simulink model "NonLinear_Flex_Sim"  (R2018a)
settings: Solver=ode3  StartTime=0.0  StopTime=10000  FixedStep=Ts  MaxStep=0.5  RelTol=1e-3  EnableMultiTasking=on
InitFcn:
  | run
StopFcn:
  | pl
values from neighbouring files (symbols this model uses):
  Cw2b = [ 0,          0,          0    [run.m]
  d2r = pi/180    (= 0.0174532925199)    [run.m]    (also in runf.m; orbitic.m; Quan.m)
  Hco = [Hy0, 0, 0]'    [run.m]
  ini = [wb0; atto; Hco]    [run.m]
  Kq1 = I22*ww^2 - 3*wo2*(I11-I33)    [run.m]
  Kq2 = 2*I22*zet*ww    [run.m]
  Kqi = 0.0005    [run.m]
  Kr1 = (0.1*I11*I33*zet^2/Hy0) - sqrt( ((0.01^zet^4*I11^2*I33^2)/Hy0^2)+(4*I11*I33*zet^2) )    [run.m]
  Kr2 = 0.05*Kr1    [run.m]
  Kr3 = 0.04*zet*(Kr2-Hy0) * sqrt(abs(Hy0/(I11*I33)))    [run.m]
  nt = 7    [run.m]    (also in runf.m)
  Tmax = 0.05    [run.m]
  Ts = 0.001    [run.m]    (also in runf.m = 0.0005)
  wb0 = [0.0, -wo, 0.0]'    [run.m]
  wo = Worb    [run.m]
  wr0 = [-500.0, 0.0, 0.0]    [run.m]
undefined symbols (not defined in the file or in its folder): Avf, Bvf, Cvf, den, DiscIntNeverNeededParam, Dvf, Mode_Switch, num, Phase_Plane, RW_Steering, Spacecraft_Dynamics, Wheel_Dynamics
libraries: simulink x4

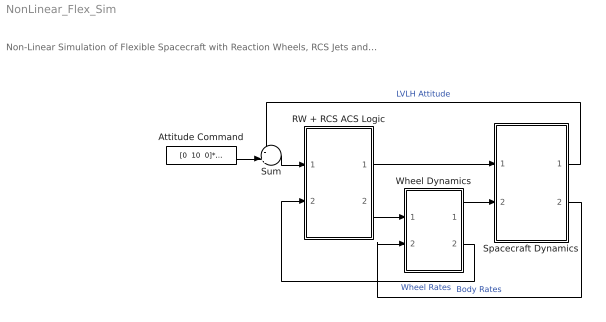
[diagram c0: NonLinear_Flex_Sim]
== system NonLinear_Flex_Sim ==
  note: Non-Linear Simulation of Flexible Spacecraft with Reaction Wheels, RCS Jets and Momentum Bias
  Attitude Command : Constant  Value="[0  10  0]*d2r"
  RW + RCS ACS Logic : Subsystem
  Spacecraft Dynamics : Subsystem
  Sum : Sum  Inputs=-+|
  Wheel Dynamics : Subsystem
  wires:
  Attitude Command/1 -> Sum/2
  Sum/1 -> RW + RCS ACS Logic/1(atter)
  Wheel Dynamics/2(wr) -> RW + RCS ACS Logic/2(wr(i))  "Wheel Rates"
  RW + RCS ACS Logic/2(Trwi) -> Wheel Dynamics/1(Twi)
  Spacecraft Dynamics/1(atti) -> Sum/1  "LVLH Attitude"
  Spacecraft Dynamics/2(wb) -> Wheel Dynamics/2(wb)  "Body Rates"
  RW + RCS ACS Logic/1(Frcs) -> Spacecraft Dynamics/1(Frcs)
  Wheel Dynamics/1(Tcb) -> Spacecraft Dynamics/2(Trwa)

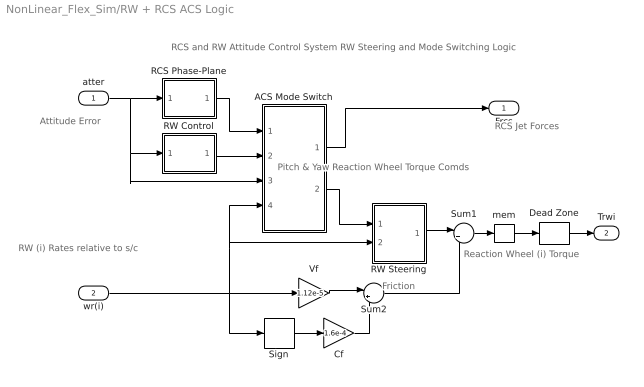
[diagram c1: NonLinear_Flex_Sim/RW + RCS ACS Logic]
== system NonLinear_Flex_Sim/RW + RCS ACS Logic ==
  note: Reaction Wheel (i) Torque
  note: RW (i) Rates relative to s/c
  note: Attitude Error
  note: Pitch & Yaw Reaction Wheel Torque Comds
  note: Friction
  note: RCS Jet Forces
  note: RCS and RW Attitude Control System RW Steering and Mode Switching Logic
  atter : Inport
  wr(i) : Inport  Port=2
  ACS Mode Switch : Subsystem
  Cf : Gain  Gain=1.6e-4
  Dead Zone : DeadZone  LowerValue=-[1, 1, 1]*Tmax/1000  UpperValue=[1 1 1]*Tmax/1000
  RCS Phase-Plane : Subsystem
  RW Control : Subsystem
  RW Steering : Subsystem
  Sign : Signum
  Sum1 : Sum  Inputs=|+-
  Sum2 : Sum  Inputs=|++
  Vf : Gain  Gain=1.12e-5
  mem : Memory  InheritSampleTime=on
  Frcs : Outport
  Trwi : Outport  Port=2
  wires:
  atter/1 -> RCS Phase-Plane/1(atter), ACS Mode Switch/3(atter), RW Control/1(atti)
  RW Control/1(Tc) -> ACS Mode Switch/2(Trw)
  RCS Phase-Plane/1(f(nt)) -> ACS Mode Switch/1(Frcs)
  ACS Mode Switch/2(" Trw") -> RW Steering/1(Trwc)
  ACS Mode Switch/1(" Frcs") -> Frcs/1
  RW Steering/1(Twic) -> Sum1/1
  Sum1/1 -> mem/1
  Dead Zone/1 -> Trwi/1
  Cf/1 -> Sum2/2
  Vf/1 -> Sum2/1
  Sign/1 -> Cf/1
  Sum2/1 -> Sum1/2
  mem/1 -> Dead Zone/1
  wr(i)/1 -> ACS Mode Switch/4(wr(i)), RW Steering/2(wr(1)), Sign/1, Vf/1

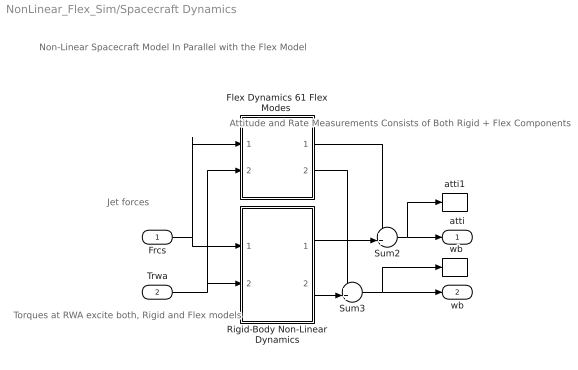
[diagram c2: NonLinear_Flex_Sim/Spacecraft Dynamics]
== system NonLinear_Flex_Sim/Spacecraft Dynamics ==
  note: Non-Linear Spacecraft Model In Parallel with the Flex Model
  note: Torques at RWA excite both, Rigid and Flex models
  note: Jet forces
  note: Attitude and Rate Measurements Consists of Both Rigid + Flex Components
  Frcs : Inport
  Trwa : Inport  Port=2
  "  wb " : ToWorkspace  VariableName=wb  SampleTime=-1
  "Flex Dynamics 61 Flex Modes " : Subsystem
  Rigid-Body Non-Linear Dynamics : Subsystem
  Sum2 : Sum  Inputs=++|
  Sum3 : Sum  Inputs=++|
  atti1 : ToWorkspace  VariableName=atti  SampleTime=-1
  atti : Outport
  wb : Outport  Port=2
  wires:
  Frcs/1 -> "Flex Dynamics 61 Flex Modes "/1(Frcs), Rigid-Body Non-Linear Dynamics/1(Frcs)
  Trwa/1 -> "Flex Dynamics 61 Flex Modes "/2(Trwi), Rigid-Body Non-Linear Dynamics/2(Tcb)
  "Flex Dynamics 61 Flex Modes "/1(att-flx) -> Sum2/1
  Rigid-Body Non-Linear Dynamics/1(atti) -> Sum2/2
  Rigid-Body Non-Linear Dynamics/2(wbr) -> Sum3/2
  "Flex Dynamics 61 Flex Modes "/2(wb-flx) -> Sum3/1
  Sum2/1 -> atti/1, atti1/1
  Sum3/1 -> wb/1, "  wb "/1

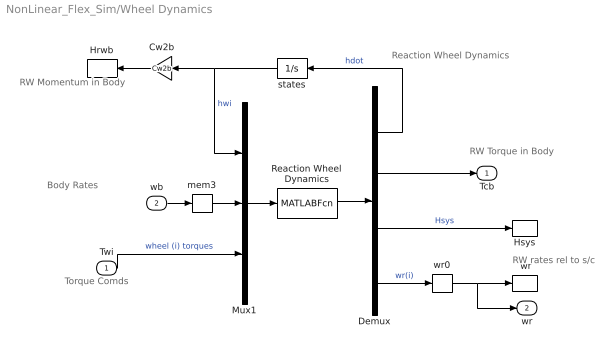
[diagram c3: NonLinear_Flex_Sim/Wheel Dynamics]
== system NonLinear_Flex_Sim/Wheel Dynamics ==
  note: Reaction Wheel Dynamics
  note: Body Rates
  note: RW Torque in Body
  note: RW rates rel to s/c
  note: Torque Comds
  note: RW Momentum in Body
  Twi : Inport
  wb : Inport  Port=2
  " wr" : ToWorkspace  VariableName=wr  SampleTime=-1
  Cw2b : Gain  Gain=Cw2b  Multiplication=Matrix(K*u)
  Demux : Demux  Outputs=[3, 3, 3, 3]
  Hrwb : ToWorkspace  VariableName=Hrwb  SampleTime=-1
  Hsys : ToWorkspace  VariableName=Hsys  SampleTime=-1
  Mux1 : Mux  Inputs=[3, 3, 3]
  Reaction Wheel Dynamics : MATLABFcn  MATLABFcn=Wheel_Dynamics( u(1:3), u(4:6), u(7:9) )  OutputDimensions=3+3+3+3
  mem3 : Memory  InitialCondition=wb0  InheritSampleTime=on
  states : Integrator  InitialCondition=Hco
  wr0 : Memory  InitialCondition=wr0  InheritSampleTime=on
  Tcb : Outport
  wr : Outport  Port=2
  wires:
  states/1 -> Cw2b/1, Mux1/1  "hwi"
  Cw2b/1 -> Hrwb/1
  Demux/1 -> states/1  "hdot"
  Demux/3 -> Hsys/1  "Hsys"
  Demux/4 -> wr0/1  "wr(i)"
  wb/1 -> mem3/1
  Mux1/1 -> Reaction Wheel Dynamics/1
  Reaction Wheel Dynamics/1 -> Demux/1
  Demux/2 -> Tcb/1
  Twi/1 -> Mux1/3  "wheel (i) torques"
  mem3/1 -> Mux1/2
  wr0/1 -> " wr"/1, wr/1

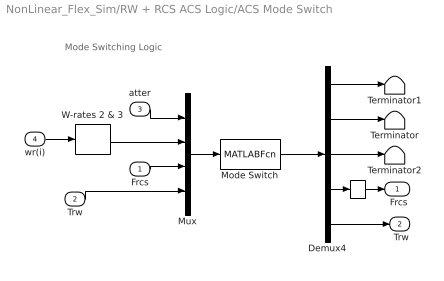
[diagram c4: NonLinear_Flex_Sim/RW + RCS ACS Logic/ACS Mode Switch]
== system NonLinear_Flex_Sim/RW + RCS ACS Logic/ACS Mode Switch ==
  note: Mode Switching Logic
  Frcs : Inport
  Trw : Inport  Port=2
  atter : Inport  Port=3
  wr(i) : Inport  Port=4
  "   " : Memory
  Demux4 : Demux  Outputs="[1 1 1 nt  2]"
  Mode Switch : MATLABFcn  MATLABFcn=Mode_Switch( u(1:3), u(4:5), u(6:5+nt), u(6+nt:7+nt) )  OutputDimensions=3+nt+2
  Mux : Mux  Inputs="[3  2  nt 2]"
  Terminator : Terminator
  Terminator1 : Terminator
  Terminator2 : Terminator
  W-rates 2 & 3 : Selector  InputPortWidth=3  IndexOptions=Index vector (dialog)  Indices="[2  3]"  OutputSizes=1
  " Frcs" : Outport
  " Trw" : Outport  Port=2
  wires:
  atter/1 -> Mux/1
  Mux/1 -> Mode Switch/1
  wr(i)/1 -> W-rates 2 & 3/1
  Frcs/1 -> Mux/3
  Trw/1 -> Mux/4
  Mode Switch/1 -> Demux4/1
  Demux4/4 -> "   "/1
  Demux4/5 -> " Trw"/1
  "   "/1 -> " Frcs"/1
  W-rates 2 & 3/1 -> Mux/2
  Demux4/1 -> Terminator1/1
  Demux4/2 -> Terminator/1
  Demux4/3 -> Terminator2/1

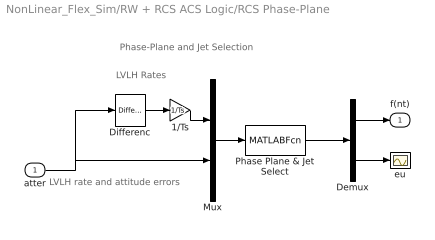
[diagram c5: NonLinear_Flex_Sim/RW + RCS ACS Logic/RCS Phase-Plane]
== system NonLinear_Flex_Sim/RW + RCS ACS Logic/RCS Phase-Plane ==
  note: LVLH rate and attitude errors
  note: LVLH Rates
  note: Phase-Plane and Jet Selection
  atter : Inport
  1/Ts : Gain  Gain=1/Ts
  Demux : Demux  Outputs=[nt, 3]
  Differenc : simulink/Discrete/Difference  ICPrevInput=0.0  InputProcessing=Inherited  OutMin=[]  OutMax=[]  OutDataType=sfix(16)  OutScaling=2^-10  DoSatur=off
  Mux : Mux  Inputs="[3  3]"
  Phase Plane & Jet Select : MATLABFcn  MATLABFcn=Phase_Plane( u(1:3), u(4:6) )  OutputDimensions=nt + 3
  eu : Scope
  f(nt) : Outport
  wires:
  atter/1 -> Mux/2, Differenc/1
  1/Ts/1 -> Mux/1
  Demux/2 -> eu/1
  Demux/1 -> f(nt)/1
  Phase Plane & Jet Select/1 -> Demux/1
  Mux/1 -> Phase Plane & Jet Select/1
  Differenc/1 -> 1/Ts/1

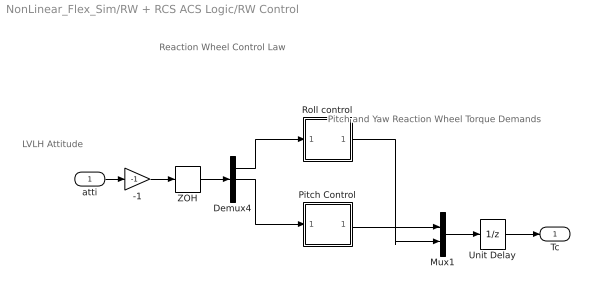
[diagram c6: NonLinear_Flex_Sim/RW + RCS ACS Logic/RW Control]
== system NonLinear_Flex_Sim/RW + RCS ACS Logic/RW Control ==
  note: Pitch and Yaw Reaction Wheel Torque Demands
  note: LVLH Attitude
  note: Reaction Wheel Control Law
  atti : Inport
  -1 : Gain  Gain=-1
  Demux4 : Demux  Outputs=3
  Mux1 : Mux  Inputs=2
  Pitch Control : Subsystem
  Roll control : Subsystem
  Unit Delay : UnitDelay  SampleTime=-1
  ZOH : ZeroOrderHold  SampleTime=Ts
  Tc : Outport
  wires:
  Demux4/1 -> Roll control/1(phi)
  Pitch Control/1(Tcy) -> Mux1/1
  Demux4/2 -> Pitch Control/1(the)
  atti/1 -> -1/1
  Roll control/1(Tcz) -> Mux1/2
  Mux1/1 -> Unit Delay/1
  ZOH/1 -> Demux4/1
  -1/1 -> ZOH/1
  Unit Delay/1 -> Tc/1

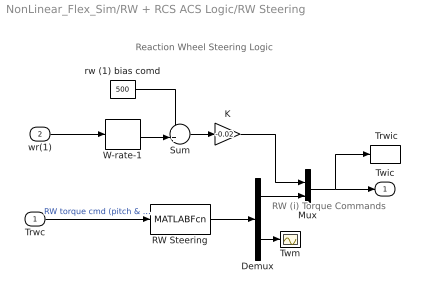
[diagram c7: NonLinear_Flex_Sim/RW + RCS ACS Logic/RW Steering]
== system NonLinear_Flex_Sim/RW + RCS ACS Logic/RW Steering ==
  note: RW (i) Torque Commands
  note: Reaction Wheel Steering Logic
  Trwc : Inport
  wr(1) : Inport  Port=2
  " Trwic" : ToWorkspace  VariableName=Twic  SampleTime=-1
  Demux : Demux  Outputs=[2, 1]
  K : Gain  Gain=-0.02
  Mux : Mux  Inputs=[1,2]
  RW Steering : MATLABFcn  MATLABFcn=RW_Steering( u(1:2) )  OutputDimensions=3
  Sum : Sum  Inputs=++|
  Twm : Scope
  W-rate-1 : Selector  InputPortWidth=3  IndexOptions=Index vector (dialog)  Indices=[1]  OutputSizes=1
  rw (1) bias comd : Constant  Value=500
  Twic : Outport
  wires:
  Demux/2 -> Twm/1
  Demux/1 -> Mux/2
  RW Steering/1 -> Demux/1
  Trwc/1 -> RW Steering/1  "RW torque cmd (pitch & yaw)"
  wr(1)/1 -> W-rate-1/1
  Sum/1 -> K/1
  rw (1) bias comd/1 -> Sum/1
  W-rate-1/1 -> Sum/2
  K/1 -> Mux/1
  Mux/1 -> Twic/1, " Trwic"/1

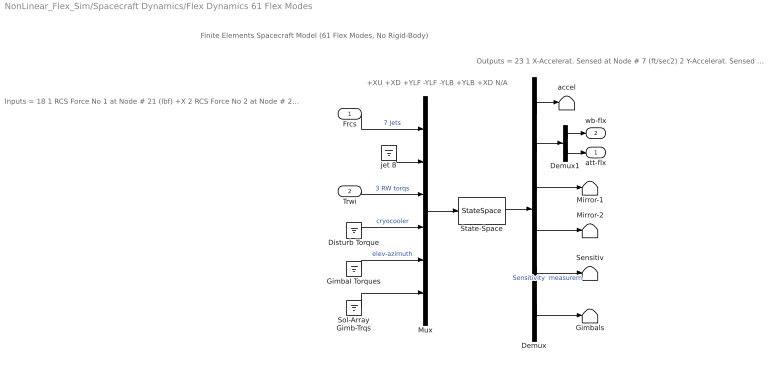
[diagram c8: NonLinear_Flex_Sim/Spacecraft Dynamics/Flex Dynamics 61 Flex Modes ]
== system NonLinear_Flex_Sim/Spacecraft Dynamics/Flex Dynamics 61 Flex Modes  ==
  note: +XU +XD +YLF -YLF -YLB +YLB +XD N/A
  note: Outputs = 23 1 X-Accelerat. Sensed at Node # 7 (ft/sec2) 2 Y-Accelerat. Sensed at Node # 7 (ft/sec2) 3 X-Rot. Rate Sensed at Node # 6 (radian) 4 Y-Rot. Rate Sensed at Node # 6 (radian) 5 Z-Rot. Rate Sensed at Node # 6 (radian) 6 X-Rotation Sensed at Node # 6 (radian) 7 Y-Rotation Sensed at Node # 6 (radian) 8 Z-Rotation Sensed at Node # 6 (radian) 9 Y-Rotation Mirror at Node # 9 (radian) 10 Z-Rotation Mirror at Node # 9 (radian) 11 Y-Rotation Instrum-2 Node # 10 (radian) 12 Z-Rotation Instrum-2 Node # 10 (radian) 13 X-Rotation Instrum-3 Node # 11 (radian) 14 Y-Rotation Instrum-4 Node # 12 (radian) 15 Z-Rotation Instrum-5 Node # 13 (radian) 16 Rotation Angle at Elevati Gimbal No 1 17 Rotation Rate at Elevati Gimbal No 1 18 Rotation Angle at Azimuth Gimbal No 2 19 Rotation Rate at Azimuth Gimbal No 2 20 Rotation Angle at Rght SA Gimbal No 3 21 Rotation Rate at Rght SA Gimbal No 3 22 Rotation Angle at Left SA Gimbal No 4 23 Rotation Rate at Left SA Gimbal No 4
  note: Inputs = 18 1 RCS Force No 1 at Node # 21 (lbf) +X 2 RCS Force No 2 at Node # 22 (lbf) +X 3 RCS Force No 3 at Node # 23 (lbf) +Y 4 RCS Force No 4 at Node # 24 (lbf) -Y 5 RCS Force No 5 at Node # 25 (lbf) -Y 6 RCS Force No 6 at Node # 26 (lbf) +Y 7 RCS Force No 7 at Node # 27 (lbf) +X 8 RCS Force No 8 at Node # 28 (lbf) +X 9 RW Torque No 1 at Node # 17 (ft-lb) roll 10 RW Torque No 2 at Node # 18 (ft-lb) ptch 11 RW Torque No 3 at Node # 19 (ft-lb) yaw 12 Dist Trque No 4 at Node # 8 (ft-lb) roll 13 Dist Trque No 5 at Node # 8 (ft-lb) ptch 14 Dist Trque No 6 at Node # 8 (ft-lb) yaw 15 Elevation Trqu at Gimbal No 1 (ft-lb) 16 Azimuth Torque at Gimbal No 2 (ft-lb) 17 Rght SA Torque at Gimbal No 3 (ft-lb) 18 Left SA Torque at Gimbal No 4 (ft-lb)
  note: Finite Elements Spacecraft Model (61 Flex Modes, No Rigid-Body)
  Frcs : Inport
  Trwi : Inport  Port=2
  Demux : Demux  Outputs="[2, 6, 2,2,3,  8]"
  Demux1 : Demux  Outputs=[3, 3]
  Disturb Torque : Ground
  Gimbal Torques : Ground
  Gimbals : Terminator
  Mirror-1 : Terminator
  Mirror-2 : Terminator
  Mux : Mux  Inputs=[7,1,3,3,2,2]
  Sensitiv : Terminator
  Sol-Array Gimb-Trqs : Ground
  State-Space : StateSpace  A=Avf  B=Bvf  C=Cvf  D=Dvf  InitialCondition=0
  accel : Terminator
  jet 8 : Ground
  att-flx : Outport
  wb-flx : Outport  Port=2
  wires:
  Demux1/2 -> att-flx/1
  Demux/4 -> Mirror-2/1
  Demux/3 -> Mirror-1/1
  Demux/5 -> Sensitiv/1  "Sensitivity  measurem"
  Sol-Array Gimb-Trqs/1 -> Mux/6
  Disturb Torque/1 -> Mux/4  "cryocooler"
  Trwi/1 -> Mux/3  "3 RW torqs"
  jet 8/1 -> Mux/2
  Frcs/1 -> Mux/1  "7 Jets"
  Mux/1 -> State-Space/1
  Demux1/1 -> wb-flx/1
  Demux/2 -> Demux1/1
  State-Space/1 -> Demux/1
  Demux/1 -> accel/1
  Gimbal Torques/1 -> Mux/5  "elev-azimuth"
  Demux/6 -> Gimbals/1

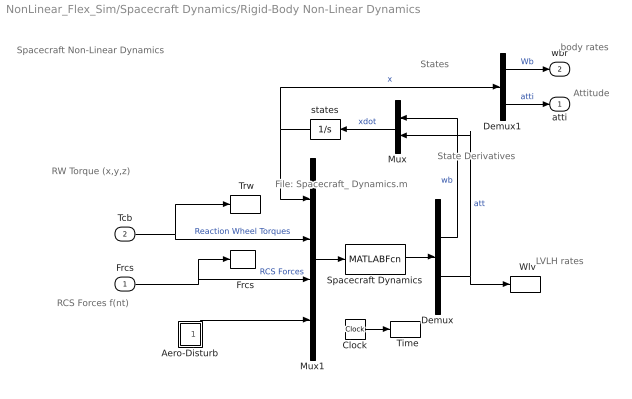
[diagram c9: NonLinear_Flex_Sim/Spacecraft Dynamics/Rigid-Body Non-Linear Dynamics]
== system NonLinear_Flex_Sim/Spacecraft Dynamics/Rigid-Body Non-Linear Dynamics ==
  note: Spacecraft Non-Linear Dynamics
  note: State Derivatives
  note: body rates
  note: RCS Forces f(nt)
  note: States
  note: RW Torque (x,y,z)
  note: LVLH rates
  note: Attitude
  note: File: Spacecraft_ Dynamics.m
  Frcs : Inport  PortDimensions=nt
  Tcb : Inport  Port=2
  "  Frcs" : ToWorkspace  VariableName=Frcs  SampleTime=-1
  "  Time" : ToWorkspace  VariableName=time  SampleTime=-1
  "  Wlv" : ToWorkspace  VariableName=wlv  SampleTime=-1
  " Trw" : ToWorkspace  VariableName=Trwb  SampleTime=-1
  Aero-Disturb : Subsystem
  Clock : Clock
  Demux : Demux  Outputs=[3,3]
  Demux1 : Demux  Outputs=[3,3]
  Mux : Mux  Inputs=[3,3]
  Mux1 : Mux  Inputs=[6, 3, nt, 3]
  Spacecraft Dynamics : MATLABFcn  MATLABFcn=Spacecraft_Dynamics( u(1:6), u(7:9), u(10:9+nt), u(10+nt:12+nt) )  OutputDimensions=6
  states : Integrator  InitialCondition=ini
  atti : Outport
  wbr : Outport  Port=2
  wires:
  Mux/1 -> states/1  "xdot"
  Clock/1 -> "  Time"/1
  Frcs/1 -> "  Frcs"/1, Mux1/3  "RCS Forces"
  states/1 -> Demux1/1, Mux1/1  "x"
  Demux/2 -> Mux/2, "  Wlv"/1  "att"
  Demux/1 -> Mux/1  "wb"
  Mux1/1 -> Spacecraft Dynamics/1
  Spacecraft Dynamics/1 -> Demux/1
  Demux1/1 -> wbr/1  "Wb"
  Demux1/2 -> atti/1  "atti"
  Tcb/1 -> Mux1/2, " Trw"/1  "Reaction Wheel Torques"
  Aero-Disturb/1(Td) -> Mux1/4

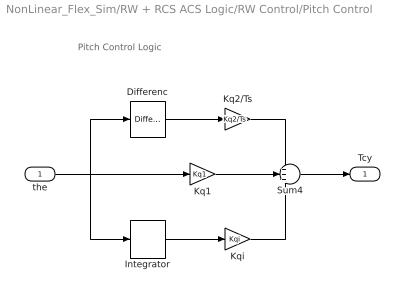
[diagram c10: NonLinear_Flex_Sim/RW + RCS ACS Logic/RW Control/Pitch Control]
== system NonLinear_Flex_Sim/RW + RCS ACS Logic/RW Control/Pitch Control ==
  note: Pitch Control Logic
  the : Inport
  Differenc : simulink/Discrete/Difference  ICPrevInput=-0.1757  InputProcessing=Inherited  OutMin=[]  OutMax=[]  OutDataType=sfix(16)  OutScaling=2^-10  DoSatur=off
  Integrator : DiscreteIntegrator  SampleTime=Ts  ICPrevOutput=DiscIntNeverNeededParam  ICPrevScaledInput=DiscIntNeverNeededParam
  Kq1 : Gain  Gain=Kq1
  Kq2/Ts : Gain  Gain=Kq2/Ts
  Kqi : Gain  Gain=Kqi
  Sum4 : Sum  Inputs=+++
  Tcy : Outport
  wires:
  Kq1/1 -> Sum4/2
  Sum4/1 -> Tcy/1
  the/1 -> Kq1/1, Differenc/1, Integrator/1
  Kqi/1 -> Sum4/3
  Integrator/1 -> Kqi/1
  Differenc/1 -> Kq2/Ts/1
  Kq2/Ts/1 -> Sum4/1

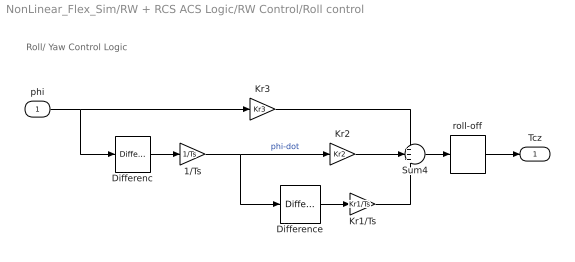
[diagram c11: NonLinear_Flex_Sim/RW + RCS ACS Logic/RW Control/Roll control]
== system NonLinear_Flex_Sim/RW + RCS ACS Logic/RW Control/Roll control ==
  note: Roll/ Yaw Control Logic
  phi : Inport
  1/Ts : Gain  Gain=1/Ts
  Differenc : simulink/Discrete/Difference  ICPrevInput=0  InputProcessing=Inherited  OutMin=[]  OutMax=[]  OutDataType=sfix(16)  OutScaling=2^-10  DoSatur=off
  Difference : simulink/Discrete/Difference  ICPrevInput=0.0  InputProcessing=Inherited  OutMin=[]  OutMax=[]  OutDataType=sfix(16)  OutScaling=2^-10  DoSatur=off
  Kr1/Ts : Gain  Gain=Kr1/Ts
  Kr2 : Gain  Gain=Kr2
  Kr3 : Gain  Gain=Kr3
  Sum4 : Sum  Inputs=+++
  roll-off : DiscreteTransferFcn  Numerator=[num]  Denominator=[den]  SampleTime=Ts
  Tcz : Outport
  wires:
  Kr3/1 -> Sum4/1
  Kr2/1 -> Sum4/2
  Kr1/Ts/1 -> Sum4/3
  phi/1 -> Kr3/1, Differenc/1
  Sum4/1 -> roll-off/1
  Difference/1 -> Kr1/Ts/1
  Differenc/1 -> 1/Ts/1
  1/Ts/1 -> Kr2/1, Difference/1  "phi-dot"
  roll-off/1 -> Tcz/1

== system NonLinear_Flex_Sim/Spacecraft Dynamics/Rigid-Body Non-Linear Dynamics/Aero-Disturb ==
  note: Aerodynamic Disturbance Torques
  30 : Gain  Gain=30
  Disturb Trq1 : Sin  Amplitude="[0.0,  1.2,  0.4]*0.0001"  Bias="[0.0,  0.6,  0.2]*0.0001"  Frequency=[wo, wo, wo]  SampleTime=0
  Disturb Trq2 : Sin  Amplitude=[0, 1.2, 1]*0.0001  Bias="[0  0.2  0.1]*0.0001"  Frequency=[wo, wo, wo]*2  SampleTime=0
  Sum2 : Sum  Inputs=+|+
  "Td " : ToWorkspace  VariableName=Td  SampleTime=-1
  Td : Outport
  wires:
  30/1 -> "Td "/1, Td/1
  Disturb Trq2/1 -> Sum2/2  "2*wo"
  Sum2/1 -> 30/1
  Disturb Trq1/1 -> Sum2/1  "wo"
